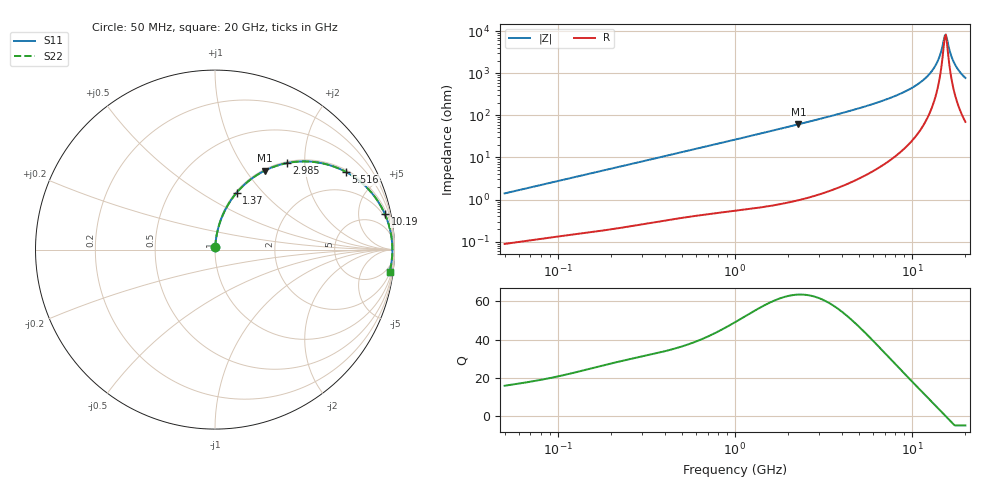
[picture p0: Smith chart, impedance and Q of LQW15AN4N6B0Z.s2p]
!Murata Part Number: LQW15AN4N6B0Z
!These Parameters are Measured in Series Mode Connection
!  o--[Z]--o
!Port1  Port2
!  o-------o
!Freq. Start=50[MHz] Stop=20[GHz], 401[Steps]
# Hz S RI R 50
!Freq.(Hz) S11(Real) S11(Imag) S21(Real) S21(Imag) S12(Real) S12(Imag) S22(Real) S22(Imag)
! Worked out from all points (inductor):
!   401 points, 50 MHz to 20 GHz, reference 50 ohm
!   read as one part in series: L = 4.42 nH near 51.52 MHz
!   highest Q = 63.5 at 2.279 GHz (marker M1), where L = 4.28 nH
!   self-resonance near 15.27 GHz
!   S11 on the Smith chart (normalised r, x): 50 MHz: 1.00, +0.03; 1.37 GHz: 1.01, +0.73; 2.985 GHz: 1.03, +1.63; 5.516 GHz: 1.08, +3.32; 10.19 GHz: 1.55, +9.46; 20 GHz: 2, -15
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5e7  0.00108 0.014  0.9989 -0.014  0.9989 -0.014  0.00108 0.014
1.364002e8  0.00295 0.0371  0.997 -0.0371  0.997 -0.0371  0.00295 0.0371
3.721004e8  0.0128 0.0982  0.9872 -0.0982  0.9872 -0.0982  0.0128 0.0982
1e9  0.0701 0.2454  0.9299 -0.2454  0.9299 -0.2454  0.0701 0.2454
1.369645e9  0.1212 0.3177  0.8788 -0.3177  0.8788 -0.3177  0.1212 0.3177
2.279204e9  0.2762 0.4393  0.7238 -0.4393  0.7238 -0.4393  0.2762 0.4393
2.728004e9  0.3563 0.471  0.6437 -0.471  0.6437 -0.471  0.3563 0.471
2.98453e9  0.4007 0.482  0.5993 -0.482  0.5993 -0.482  0.4007 0.482
5.515528e9  0.7292 0.4329  0.2708 -0.4329  0.2708 -0.4329  0.7292 0.4329
7.442007e9  0.8583 0.3327  0.1417 -0.3327  0.1417 -0.3327  0.8583 0.3327
1.019291e10  0.9468 0.1971  0.0532 -0.1971  0.0532 -0.1971  0.9468 0.1971
1.183995e10  0.9714 0.1272  0.0286 -0.1272  0.0286 -0.1272  0.9714 0.1272
1.314879e10  0.9821 0.0773  0.0179 -0.0773  0.0179 -0.0773  0.9821 0.0773
1.396067e10  0.9858 0.0486  0.0142 -0.0486  0.0142 -0.0486  0.9858 0.0486
1.438523e10  0.9871 0.0342  0.0129 -0.0342  0.0129 -0.0342  0.9871 0.0342
1.504638e10  0.9881 0.0126  0.0119 -0.0126  0.0119 -0.0126  0.9881 0.0126
1.550395e10  0.9883 -0.00187  0.0117 0.00187  0.0117 0.00187  0.9883 -0.00187
1.573793e10  0.9882 -0.00908  0.0118 0.00908  0.0118 0.00908  0.9882 -0.00908
1.670968e10  0.9869 -0.0379  0.0131 0.0379  0.0131 0.0379  0.9869 -0.0379
1.747767e10  0.9848 -0.0595  0.0152 0.0595  0.0152 0.0595  0.9848 -0.0595
1.88369e10  0.9791 -0.0954  0.0209 0.0954  0.0209 0.0954  0.9791 -0.0954
2e10  0.9726 -0.1239  0.0274 0.1239  0.0274 0.1239  0.9726 -0.1239
